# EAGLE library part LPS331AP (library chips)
IC PRESSURE SENSOR PIEZO 16HCLGA
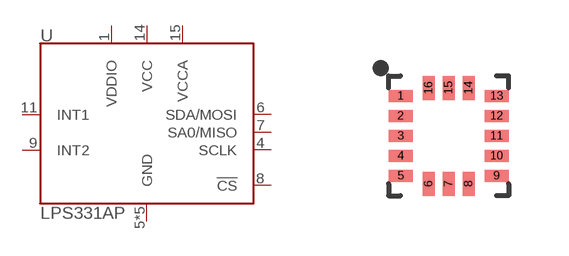
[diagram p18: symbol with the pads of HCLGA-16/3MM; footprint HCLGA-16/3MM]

Designator prefix U

## LPS331AP (DIGIKEY: 497-12927-1-ND)  [HCLGA-16/3MM]
1  VDDIO
4  SCLK
5  GND
6  SDA/MOSI
7  SA0/MISO
8  !CS
9  INT2
10  GND
11  INT1
12  GND
13  GND
14  VCC
15  VCCA
16  GND

## Footprint HCLGA-16/3MM (pad centres in mm)
smd 0.6 x 0.3: 1 -1.2,1; 2 -1.2,0.5; 3 -1.2,0; 4 -1.2,-0.5; 5 -1.2,-1; 9 1.2,-1; 10 1.2,-0.5; 11 1.2,0; 12 1.2,0.5; 13 1.2,1
smd 0.3 x 0.6: 6 -0.5,-1.2; 7 0,-1.2; 8 0.5,-1.2; 14 0.5,1.2; 15 0,1.2; 16 -0.5,1.2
